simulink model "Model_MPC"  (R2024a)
settings: Solver=VariableStepAuto  StartTime=0.0  StopTime=10.0  RelTol=1e-3
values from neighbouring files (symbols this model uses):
  A_f = 2.15    [main.m]    (also in prediction_longitudinal_model.m; MPC_and_plant_params.m; prediction_model_test.m; main_BW_FW.m)
  alpha = 0*pi/180    (= 0)    [main.m]    (also in prediction_longitudinal_model.m; MPC_and_plant_params.m; prediction_model_test.m; main_BW_FW.m)
  C_d = 0.33    [main.m]    (also in prediction_longitudinal_model.m; MPC_and_plant_params.m; prediction_model_test.m; main_BW_FW.m)
  default_distance = 10    [main.m]    (also in MPC_and_plant_params.m = 50)
  eff = e    [polinomial_fits.m]    (also in eff_poly.m; main.m = Efficiency/100; MPC_and_plant_params.m = Efficiency/100; main_BW_FW.m = Efficiency/100)
  f_0 = 4.5*1e-3    (= 0.0045)    [main.m]    (also in prediction_longitudinal_model.m; MPC_and_plant_params.m; prediction_model_test.m; main_BW_FW.m)
  g = 9.81    [main.m]    (also in prediction_longitudinal_model.m; MPC_and_plant_params.m; prediction_model_test.m; main_BW_FW.m)
  h = 0.3    [main.m]    (also in prediction_longitudinal_model.m; MPC_and_plant_params.m = 2; main_BW_FW.m)
  K = nmpc_design_4b(par)    [main.m]
  lambda = 0.5    [main.m]    (also in MPC_and_plant_params.m)
  M_veh = 1400    [main.m]    (also in prediction_longitudinal_model.m; MPC_and_plant_params.m; prediction_model_test.m; main_BW_FW.m)
  max_acc = 2    [main.m]    (also in MPC_and_plant_params.m)
  min_acc = -3    [main.m]    (also in MPC_and_plant_params.m)
  N_p = 1    [main.m]    (also in prediction_longitudinal_model.m; MPC_and_plant_params.m; prediction_model_test.m; main_BW_FW.m)
  N_s = 108    [main.m]    (also in prediction_longitudinal_model.m; MPC_and_plant_params.m; prediction_model_test.m; main_BW_FW.m)
  r_w = 0.3    [main.m]    (also in prediction_longitudinal_model.m; MPC_and_plant_params.m; prediction_model_test.m; main_BW_FW.m)
  ref_mode = 3    [main.m]
  rho = 1.25    [main.m]    (also in prediction_longitudinal_model.m; MPC_and_plant_params.m; prediction_model_test.m; main_BW_FW.m)
  Ro_s = F_Ro_s(SOC_vec)    [main.m]    (also in MPC_and_plant_params.m; main_BW_FW.m)
  s = tf('s')    [main.m]    (also in MPC_and_plant_params.m; polinomial_fits.m = size(Speed))
  SOC0 = 0.8    [main.m]    (also in MPC_and_plant_params.m; prediction_model_test.m; main_BW_FW.m)
  SOC_vec = linspace(0,1,500)    [main.m]    (also in MPC_and_plant_params.m; main_BW_FW.m)
  tau_gb = 9.6    [main.m]    (also in prediction_longitudinal_model.m; MPC_and_plant_params.m; prediction_model_test.m; main_BW_FW.m)
  time_gap = 3    [main.m]    (also in MPC_and_plant_params.m)
  Ts = 0.05    [main.m]    (also in MPC_and_plant_params.m)
  v0 = vehspeed(1)    [main.m]    (also in MPC_and_plant_params.m; prediction_model_test.m = 0)
  v_set = 40    [main.m]    (also in MPC_and_plant_params.m)
  verr_gain = 0.1    [main.m]    (also in MPC_and_plant_params.m)
  Voc_s = F_Voc_s(SOC_vec)    [main.m]    (also in MPC_and_plant_params.m; main_BW_FW.m)
  vx_gain = 0.5    [main.m]    (also in MPC_and_plant_params.m)
  x0 = 0    [main.m]    (also in MPC_and_plant_params.m; prediction_model_test.m)
  xerr_gain = 0.3    [main.m]    (also in MPC_and_plant_params.m)
undefined symbols (not defined in the file or in its folder): flip, m, seconds, Shaft_Torque, Speed
libraries: slpidlib x2, autolibshared x1, cstblocks x1

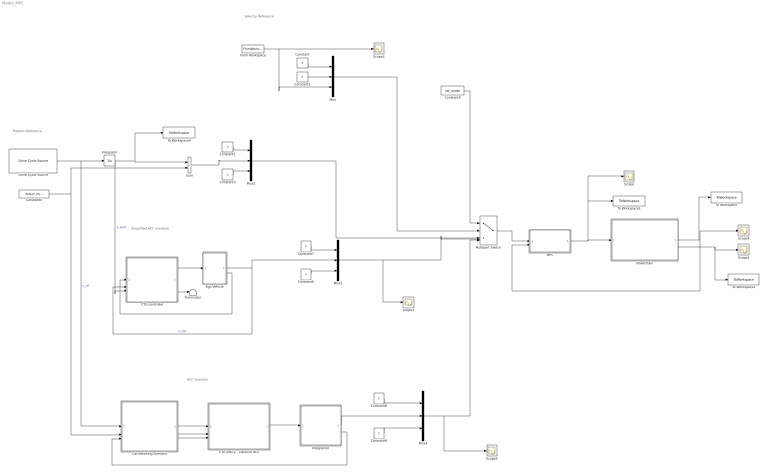
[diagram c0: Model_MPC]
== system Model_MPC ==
  note: Velocity Reference
  note: Position Reference
  note: Simplified ACC Scenario
  note: ACC Scenario
  CTG controller : Subsystem
  CTG policy - classical ACC : Subsystem  Commented=on
  Car-following Scenario : Subsystem  Commented=on
  Constant{,1..3,8..9} (6 alike) : Constant  Commented=on  Value=0
  Constant4 : Constant  Value=default_distance
  Constant5 : Constant  Value=ref_mode
  Constant6 : Constant  Value=0
  Constant7 : Constant  Value=0
  Drive Cycle Source : autolibshared/Drive Cycle Source  cycleVar=Workspace variable  wsVar=vehspeed  fileVar=cycleFTP75.mat  tfinal="1800  seconds"  cycleRepeat=off  outAccPort=off  outGearPort=off  gearList=No gear data  t_wot1=5  xdot_woto=0  xdot_wot1=30  t_wot2=20  xdot_wot2=0  t_wotend=30  srcUnit=m/s  outUnit=m/s  srcAccUnit=m/s/s  outAccUnit=m/s^2  dt=0  aMode=1  faultOption=off  velBnd=2  velBndUnit=mph  inUnit=m/s  timeBnd=1  failOption=off  stopSim=off  maxFaultCnt=10  maxFaultTime=2  maxTotFaultTime=15  traceOption=off  dtTrace=1  traceWindow=10  lastDCname=Custom Data Set  lastOutUnit=mph  lastDT=0  lastTB=1  lastSB=2  forceCalcBound=off
  Ego Vehicle : Subsystem
  From Workspace : FromWorkspace  Commented=on  VariableName=vehspeed  SampleTime=0.1  OutputAfterFinalValue=Holding final value
  Integration : Subsystem  Commented=on
  Integrator : Integrator  InitialCondition=default_distance
  MPC : Subsystem
  Multiport Switch : MultiPortSwitch  Inputs=4
  Mux : Mux  Commented=on  Inputs=3
  Mux1 : Mux  Commented=on  Inputs=3
  Mux2 : Mux  Inputs=3
  Mux3 : Mux  Commented=on  Inputs=3
  Powertrain : Subsystem
  Scope{,1..5} (6 alike) : Scope
  Sum : Sum  Commented=on  Inputs=+-
  Terminator : Terminator
  To Workspace : ToWorkspace  VariableName=X  SaveFormat=Timeseries  SampleTime=-1
  To Workspace1 : ToWorkspace  VariableName=T_EM_MPC  SaveFormat=Timeseries  SampleTime=-1
  To Workspace2 : ToWorkspace  VariableName=X_dot  SaveFormat=Timeseries  SampleTime=-1
  To Workspace4 : ToWorkspace  VariableName=pos_leading  SaveFormat=Timeseries  SampleTime=-1
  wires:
  MPC/1(u) -> Powertrain/1(T_EM), To Workspace1/1, Scope/1
  Powertrain/1(X (states)) -> To Workspace/1, MPC/2(x), Scope4/1
  Powertrain/2(X_dot) -> To Workspace2/1, Scope1/1
  From Workspace/1 -> Mux/3, Scope2/1
  Constant2/1 -> Mux/2
  Constant/1 -> Mux/1
  Drive Cycle Source/1 -> Car-following Scenario/1(lead speed [m/s]), Integrator/1  "v_ref"
  Constant1/1 -> Mux1/1
  Constant3/1 -> Mux1/3
  Integrator/1 -> To Workspace4/1, Sum/1, CTG controller/3(lead position [m])  "x_lead"
  Constant4/1 -> Car-following Scenario/2(initial distance [m]), Sum/2
  CTG controller/1(a) -> Ego Vehicle/1(a)
  Ego Vehicle/1(x) -> CTG controller/2(ego position [m]), Mux2/2  "x_ego"
  Constant7/1 -> Mux2/1
  Constant6/1 -> Mux2/3
  CTG controller/2(spacing_error) -> Terminator/1
  Multiport Switch/1 -> MPC/1(r)
  Constant5/1 -> Multiport Switch/1
  Mux1/1 -> Multiport Switch/3
  Mux2/1 -> Scope3/1, Multiport Switch/4
  Ego Vehicle/2(x_dot) -> CTG controller/1(ego speed [m/s])
  Car-following Scenario/1(d_rel) -> CTG policy - classical ACC/1(Relative Distance)
  Car-following Scenario/2(v_rel) -> CTG policy - classical ACC/2("Relative Velocity ")
  Car-following Scenario/3(v_host) -> CTG policy - classical ACC/3("Longitudinal Velocity ")
  Constant8/1 -> Mux3/1
  Constant9/1 -> Mux3/3
  Mux3/1 -> Scope5/1, Multiport Switch/5
  Sum/1 -> Mux1/2
  Mux/1 -> Multiport Switch/2
  Integration/1(x_ego) -> Mux3/2
  CTG policy - classical ACC/1(Acceleration) -> Integration/1(a)
  Integration/2(x_dot) -> Car-following Scenario/3(ego speed [m/s])

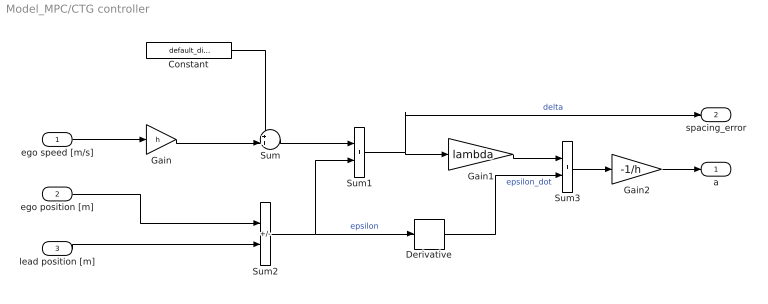
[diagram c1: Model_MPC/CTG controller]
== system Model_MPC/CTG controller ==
  ego speed [m/s] : Inport
  ego position [m] : Inport  Port=2
  lead position [m] : Inport  Port=3
  Constant : Constant  Value=default_distance
  Derivative : Derivative  CoefficientInTFapproximation=Td
  Gain : Gain  Gain=h
  Gain1 : Gain  Gain=lambda
  Gain2 : Gain  Gain=-1/h
  Sum : Sum  Inputs=++|
  Sum1 : Sum
  Sum2 : Sum  Inputs=+-
  Sum3 : Sum
  a : Outport
  spacing_error : Outport  Port=2
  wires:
  ego position [m]/1 -> Sum2/1
  lead position [m]/1 -> Sum2/2
  ego speed [m/s]/1 -> Gain/1
  Sum2/1 -> Derivative/1, Sum1/2  "epsilon"
  Sum1/1 -> spacing_error/1, Gain1/1  "delta"
  Sum3/1 -> Gain2/1
  Derivative/1 -> Sum3/2  "epsilon_dot"
  Gain1/1 -> Sum3/1
  Gain2/1 -> a/1
  Gain/1 -> Sum/2
  Sum/1 -> Sum1/1
  Constant/1 -> Sum/1

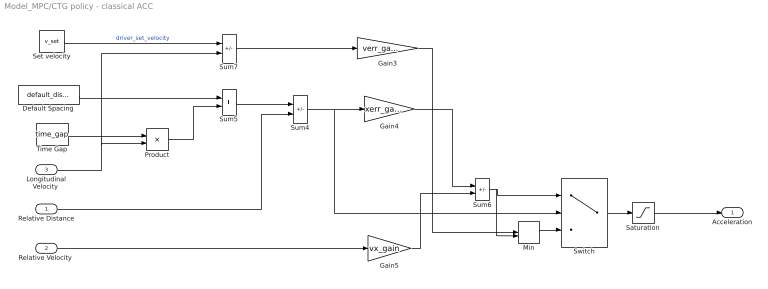
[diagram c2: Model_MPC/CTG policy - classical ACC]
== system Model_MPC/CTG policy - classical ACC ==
  Relative Distance : Inport
  "Relative Velocity " : Inport  Port=2
  "Longitudinal Velocity " : Inport  Port=3
  Default Spacing : Constant  Value=default_distance  SampleTime=Ts
  Gain3 : Gain  Gain=verr_gain
  Gain4 : Gain  Gain=xerr_gain
  Gain5 : Gain  Gain=vx_gain
  Min : MinMax  Inputs=2
  Product : Product
  Saturation : Saturate  UpperLimit=max_acc  LowerLimit=min_acc
  Set velocity : Constant  Value=v_set  SampleTime=Ts
  Sum4 : Sum  Inputs=+-
  Sum5 : Sum
  Sum6 : Sum  Inputs=-+
  Sum7 : Sum  Inputs=+-
  Switch : Switch  Criteria=u2 > Threshold
  Time Gap : Constant  Value=time_gap  SampleTime=Ts
  Acceleration : Outport  VectorParamsAs1DForOutWhenUnconnected=off
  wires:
  Sum6/1 -> Min/2, Switch/1
  Sum5/1 -> Sum4/1
  Saturation/1 -> Acceleration/1
  Min/1 -> Switch/3
  "Longitudinal Velocity "/1 -> Sum7/2, Product/2
  Set velocity/1 -> Sum7/1  "driver_set_velocity"
  Time Gap/1 -> Product/1
  Gain3/1 -> Min/1
  Relative Distance/1 -> Sum4/2
  Gain4/1 -> Sum6/1
  "Relative Velocity "/1 -> Gain5/1
  Product/1 -> Sum5/2
  Switch/1 -> Saturation/1
  Gain5/1 -> Sum6/2
  Sum7/1 -> Gain3/1
  Sum4/1 -> Switch/2, Gain4/1
  Default Spacing/1 -> Sum5/1

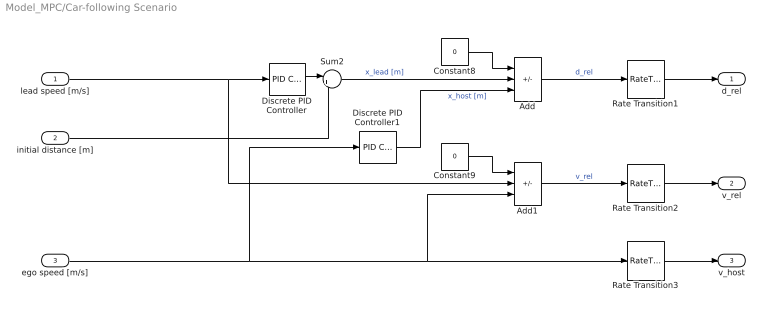
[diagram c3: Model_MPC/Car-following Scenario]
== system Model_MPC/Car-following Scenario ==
  lead speed [m/s] : Inport
  initial distance [m] : Inport  Port=2
  ego speed [m/s] : Inport  Port=3
  Add : Sum  Inputs=++-
  Add1 : Sum  Inputs=++-
  Constant8 : Constant  Value=0
  Constant9 : Constant  Value=0
  Discrete PID Controller : slpidlib/PID Controller  Controller=I  Form=Parallel  TimeDomain=Discrete-time  UseExternalTs=off  SampleTime=-1  IntegratorMethod=Forward Euler  FilterMethod=Forward Euler  ControllerParametersSource=internal  P=0  I=1  UseKiTs=off  D=0  UseExternalDerivativeSource=off  N=100  UseFilter=on  TunerSelectOption=Transfer Function Based (PID Tuner App)  InitialConditionSource=internal  InitialConditionForIntegrator=0  InitialConditionForFilter=0  DifferentiatorICPrevScaledInput=0  ExternalReset=none  TrackingMode=off  Kt=1  LimitOutput=off  SatLimitsSource=internal  UpperSaturationLimit=inf  LowerSaturationLimit=-inf  LinearizeAsGain=off  AntiWindupMode=none  Kb=1  LimitIntegrator=off  UpperIntegratorSaturationLimit=inf  LowerIntegratorSaturationLimit=-inf  POutMin=[]  POutMax=[]  IOutMin=[]  IOutMax=[]  DOutMin=[]  DOutMax=[]  NOutMin=[]  NOutMax=[]  SumOutMin=[]  SumOutMax=[]  SaturationOutMin=[]  SaturationOutMax=[]  PParamMin=[]  PParamMax=[]  IParamMin=[]  IParamMax=[]  DParamMin=[]  DParamMax=[]  NParamMin=[]  NParamMax=[]  KbParamMin=[]  KbParamMax=[]  KtParamMin=[]  KtParamMax=[]  KbOutMin=[]  KbOutMax=[]  KtOutMin=[]  KtOutMax=[]  IntegratorOutMin=[]  IntegratorOutMax=[]  FilterOutMin=[]  FilterOutMax=[]  SumI1OutMin=[]  SumI1OutMax=[]  SumI2OutMin=[]  SumI2OutMax=[]  SumI3OutMin=[]  SumI3OutMax=[]  SumI4OutMin=[]  SumI4OutMax=[]  SumDOutMin=[]  SumDOutMax=[]  DifferentiatorOutMin=[]  DifferentiatorOutMax=[]  FilterDiffOutCoefMin=[]  FilterDiffOutCoefMax=[]  ReciprocalOutMin=[]  ReciprocalOutMax=[]  SumDenOutMin=[]  SumDenOutMax=[]  SumNumOutMin=[]  SumNumOutMax=[]  DivideOutMin=[]  DivideOutMax=[]  UdiffTsProdOutMin=[]  UdiffTsProdOutMax=[]  NTsProdOutMin=[]  NTsProdOutMax=[]  UintegralTsProdOutMin=[]  UintegralTsProdOutMax=[]  UngainTsProdOutMin=[]  UngainTsProdOutMax=[]  ClampingZeroOutDataTypeStr=Inherit: Inherit via back propagation  ClampingZeroOutMin=[]  ClampingZeroOutMax=[]  FilterDenConstantOutDataTypeStr=Inherit: Inherit via back propagation  FilterDenConstantOutMin=[]  FilterDenConstantOutMax=[]  PCopyOutDataTypeStr=Inherit: Inherit via back propagation  PCopyOutMin=[]  PCopyOutMax=[]  NCopyOutDataTypeStr=Inherit: Inherit via back propagation  NCopyOutMin=[]  NCopyOutMax=[]  IntegratorContinuousStateAttributes=''  IntegratorStateMustResolveToSignalObject=off  IntegratorRTWStateStorageClass=Auto  FilterContinuousStateAttributes=''  FilterStateMustResolveToSignalObject=off  FilterRTWStateStorageClass=Auto  ParallelPVariant=Disabled  IdealPVariant=Disabled  IVariant=InternalParameters  DVariant=Disabled  IntegratorVariant=Discrete  SatVariant=Disabled  AWVariant=Passthrough  PCopyVariant=Disabled  TRVariant=Disabled  FdbkBlocksVariant=Forward  IdealPFdbkVariant=Disabled  SatFdbkVariant=Disabled  DerivativeFilterVariant=Disabled  NVariant=Disabled  NCopyVariant=Disabled_SignalSpec  FilterICVariant=Disabled  IntegratorICVariant=InternalICs  ExternalResetVariant=Disabled  TRSumVariant=Passthrough  SumFdbkVariant=Disabled  SumVariant=Passthrough_I  TsampFilterVariant=InternalTs  TsampNgainVariant=Passthrough  TsampIntegralVariant=Disabled_SignalSpec  ExternalSaturationOutDataTypeStr=Inherit: Same as second input  DerivativeSourceVariant=Disabled
  Discrete PID Controller1 : slpidlib/PID Controller  Controller=I  Form=Parallel  TimeDomain=Discrete-time  UseExternalTs=off  SampleTime=-1  IntegratorMethod=Forward Euler  FilterMethod=Forward Euler  ControllerParametersSource=internal  P=0  I=1  UseKiTs=off  D=0  UseExternalDerivativeSource=off  N=100  UseFilter=on  TunerSelectOption=Transfer Function Based (PID Tuner App)  InitialConditionSource=internal  InitialConditionForIntegrator=0  InitialConditionForFilter=0  DifferentiatorICPrevScaledInput=0  ExternalReset=none  TrackingMode=off  Kt=1  LimitOutput=off  SatLimitsSource=internal  UpperSaturationLimit=inf  LowerSaturationLimit=-inf  LinearizeAsGain=off  AntiWindupMode=none  Kb=1  LimitIntegrator=off  UpperIntegratorSaturationLimit=inf  LowerIntegratorSaturationLimit=-inf  POutMin=[]  POutMax=[]  IOutMin=[]  IOutMax=[]  DOutMin=[]  DOutMax=[]  NOutMin=[]  NOutMax=[]  SumOutMin=[]  SumOutMax=[]  SaturationOutMin=[]  SaturationOutMax=[]  PParamMin=[]  PParamMax=[]  IParamMin=[]  IParamMax=[]  DParamMin=[]  DParamMax=[]  NParamMin=[]  NParamMax=[]  KbParamMin=[]  KbParamMax=[]  KtParamMin=[]  KtParamMax=[]  KbOutMin=[]  KbOutMax=[]  KtOutMin=[]  KtOutMax=[]  IntegratorOutMin=[]  IntegratorOutMax=[]  FilterOutMin=[]  FilterOutMax=[]  SumI1OutMin=[]  SumI1OutMax=[]  SumI2OutMin=[]  SumI2OutMax=[]  SumI3OutMin=[]  SumI3OutMax=[]  SumI4OutMin=[]  SumI4OutMax=[]  SumDOutMin=[]  SumDOutMax=[]  DifferentiatorOutMin=[]  DifferentiatorOutMax=[]  FilterDiffOutCoefMin=[]  FilterDiffOutCoefMax=[]  ReciprocalOutMin=[]  ReciprocalOutMax=[]  SumDenOutMin=[]  SumDenOutMax=[]  SumNumOutMin=[]  SumNumOutMax=[]  DivideOutMin=[]  DivideOutMax=[]  UdiffTsProdOutMin=[]  UdiffTsProdOutMax=[]  NTsProdOutMin=[]  NTsProdOutMax=[]  UintegralTsProdOutMin=[]  UintegralTsProdOutMax=[]  UngainTsProdOutMin=[]  UngainTsProdOutMax=[]  ClampingZeroOutDataTypeStr=Inherit: Inherit via back propagation  ClampingZeroOutMin=[]  ClampingZeroOutMax=[]  FilterDenConstantOutDataTypeStr=Inherit: Inherit via back propagation  FilterDenConstantOutMin=[]  FilterDenConstantOutMax=[]  PCopyOutDataTypeStr=Inherit: Inherit via back propagation  PCopyOutMin=[]  PCopyOutMax=[]  NCopyOutDataTypeStr=Inherit: Inherit via back propagation  NCopyOutMin=[]  NCopyOutMax=[]  IntegratorContinuousStateAttributes=''  IntegratorStateMustResolveToSignalObject=off  IntegratorRTWStateStorageClass=Auto  FilterContinuousStateAttributes=''  FilterStateMustResolveToSignalObject=off  FilterRTWStateStorageClass=Auto  ParallelPVariant=Disabled  IdealPVariant=Disabled  IVariant=InternalParameters  DVariant=Disabled  IntegratorVariant=Discrete  SatVariant=Disabled  AWVariant=Passthrough  PCopyVariant=Disabled  TRVariant=Disabled  FdbkBlocksVariant=Forward  IdealPFdbkVariant=Disabled  SatFdbkVariant=Disabled  DerivativeFilterVariant=Disabled  NVariant=Disabled  NCopyVariant=Disabled_SignalSpec  FilterICVariant=Disabled  IntegratorICVariant=InternalICs  ExternalResetVariant=Disabled  TRSumVariant=Passthrough  SumFdbkVariant=Disabled  SumVariant=Passthrough_I  TsampFilterVariant=InternalTs  TsampNgainVariant=Passthrough  TsampIntegralVariant=Disabled_SignalSpec  ExternalSaturationOutDataTypeStr=Inherit: Same as second input  DerivativeSourceVariant=Disabled
  Rate Transition1 : RateTransition  OutPortSampleTime=0.2
  Rate Transition2 : RateTransition  OutPortSampleTime=0.2
  Rate Transition3 : RateTransition  OutPortSampleTime=0.2
  Sum2 : Sum  Inputs=|++
  d_rel : Outport
  v_rel : Outport  Port=2
  v_host : Outport  Port=3
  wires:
  initial distance [m]/1 -> Sum2/2
  Rate Transition1/1 -> d_rel/1
  Rate Transition2/1 -> v_rel/1
  ego speed [m/s]/1 -> Discrete PID Controller1/1, Add1/3, Rate Transition3/1
  Constant8/1 -> Add/1
  lead speed [m/s]/1 -> Add1/2, Discrete PID Controller/1
  Constant9/1 -> Add1/1
  Discrete PID Controller/1 -> Sum2/1
  Discrete PID Controller1/1 -> Add/3  "x_host [m]"
  Add1/1 -> Rate Transition2/1  "v_rel"
  Rate Transition3/1 -> v_host/1
  Add/1 -> Rate Transition1/1  "d_rel"
  Sum2/1 -> Add/2  "x_lead [m]"

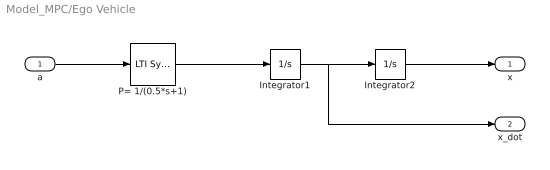
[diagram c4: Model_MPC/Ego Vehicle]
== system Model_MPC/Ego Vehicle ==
  a : Inport
  Integrator1 : Integrator
  Integrator2 : Integrator
  P= 1/(0.5*s+1) : cstblocks/LTI System  sys=P  IC=[]  PadeOrder=0
  x : Outport
  x_dot : Outport  Port=2
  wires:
  Integrator2/1 -> x/1
  Integrator1/1 -> x_dot/1, Integrator2/1
  P= 1/(0.5*s+1)/1 -> Integrator1/1
  a/1 -> P= 1/(0.5*s+1)/1

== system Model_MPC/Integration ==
  a : Inport
  Integrator1 : Integrator
  Integrator2 : Integrator
  x_ego : Outport
  x_dot : Outport  Port=2
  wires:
  Integrator2/1 -> x_ego/1  "x_ego"
  a/1 -> Integrator1/1
  Integrator1/1 -> x_dot/1, Integrator2/1

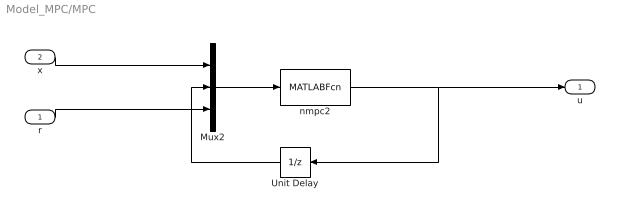
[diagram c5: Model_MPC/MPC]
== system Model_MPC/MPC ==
  r : Inport
  x : Inport  Port=2
  Mux2 : Mux  Inputs=3
  Unit Delay : UnitDelay  InitialCondition=zeros(K.nc,1)  SampleTime=K.Ts  HasFrameUpgradeWarning=on
  nmpc2 : MATLABFcn  MATLABFcn=nmpc_b2(K,u(1:K.nx),u(K.nx+1:K.nx+K.nc),u(K.nx+K.nc+1:end))  OutputDimensions=K.nc
  u : Outport
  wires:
  x/1 -> Mux2/1
  r/1 -> Mux2/3
  Unit Delay/1 -> Mux2/2
  Mux2/1 -> nmpc2/1
  nmpc2/1 -> Unit Delay/1, u/1

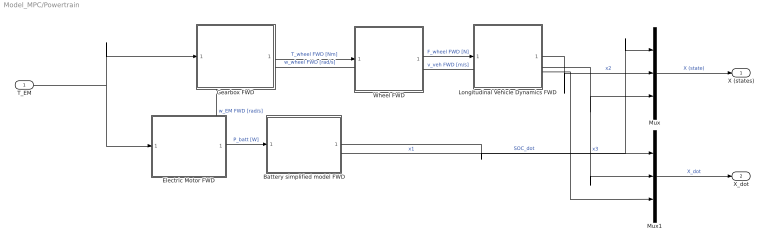
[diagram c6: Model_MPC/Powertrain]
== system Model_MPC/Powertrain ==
  T_EM : Inport
  Battery simplified model FWD : Subsystem
  Electric Motor FWD : Subsystem
  Gearbox FWD : Subsystem
  Longitudinal Vehicle Dynamics FWD : Subsystem
  Mux : Mux  Inputs=3
  Mux1 : Mux  Inputs=3
  Wheel FWD : Subsystem
  X (states) : Outport
  X_dot : Outport  Port=2
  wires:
  Battery simplified model FWD/2(SOC) -> Mux/1  "x1"
  Wheel FWD/2(w_wheel) -> Gearbox FWD/2(w_wheel)  "w_wheel FWD [rad/s]"
  Mux/1 -> X (states)/1  "X (state)"
  Gearbox FWD/1(T_wheel) -> Wheel FWD/1(T_wheel)  "T_wheel FWD [Nm]"
  Longitudinal Vehicle Dynamics FWD/2(v_veh) -> Mux1/2, Mux/3  "x3"
  Gearbox FWD/2(w_EM) -> Electric Motor FWD/2(w_EM)  "w_EM FWD [rad/s]"
  Electric Motor FWD/1(P_batt) -> Battery simplified model FWD/1(P_batt)  "P_batt [W]"
  Longitudinal Vehicle Dynamics FWD/4(v_veh1) -> Wheel FWD/2(v_veh)  "v_veh FWD [m/s]"
  Longitudinal Vehicle Dynamics FWD/1("x_veh ") -> Mux/2  "x2"
  Wheel FWD/1(F_wheel) -> Longitudinal Vehicle Dynamics FWD/1(F_trac)  "F_wheel FWD [N]"
  T_EM/1 -> Electric Motor FWD/1(T_EM), Gearbox FWD/1(T_EM)
  Battery simplified model FWD/1(SOC_dot) -> Mux1/1  "SOC_dot"
  Longitudinal Vehicle Dynamics FWD/3(a_veh) -> Mux1/3
  Mux1/1 -> X_dot/1  "X_dot"

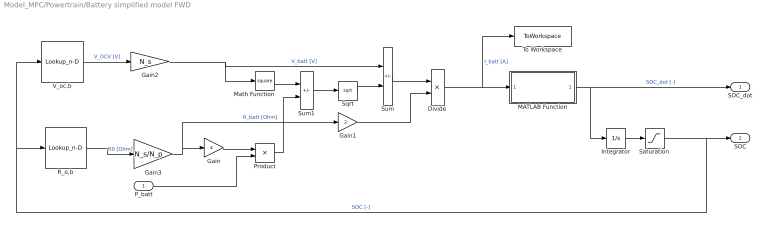
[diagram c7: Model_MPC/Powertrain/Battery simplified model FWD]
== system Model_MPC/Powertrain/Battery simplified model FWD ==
  P_batt : Inport
  Divide : Product  Inputs=*/
  Gain : Gain  Gain=4
  Gain1 : Gain  Gain=2
  Gain2 : Gain  Gain=N_s
  Gain3 : Gain  Gain=N_s/N_p
  Integrator : Integrator  InitialCondition=SOC0
  MATLAB Function : MATLAB Function  TreatAsAtomicUnit=on
  Math Function : Math  Operator=square
  Product : Product
  R_o,b : Lookup_n-D  NumberOfTableDimensions=1  BreakpointsForDimension1=SOC_vec  BreakpointsForDimension3=[5, 7]  Table=Ro_s  InternalRulePriority=Speed  RndMeth=Simplest
  Saturation : Saturate  UpperLimit=1  LowerLimit=0
  Sqrt : Sqrt
  Sum : Sum  Inputs=+-
  Sum1 : Sum  Inputs=+-
  To Workspace : ToWorkspace  VariableName=Ib_controlled  SaveFormat=Timeseries  SampleTime=-1
  V_oc,b : Lookup_n-D  NumberOfTableDimensions=1  BreakpointsForDimension1=SOC_vec  BreakpointsForDimension3=[5, 7]  Table=Voc_s  InternalRulePriority=Speed  RndMeth=Simplest
  SOC_dot : Outport
  SOC : Outport  Port=2
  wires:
  Math Function/1 -> Sum1/1
  Gain/1 -> Product/1
  Product/1 -> Sum1/2
  Sum1/1 -> Sqrt/1
  Sqrt/1 -> Sum/2
  Sum/1 -> Divide/1
  Gain1/1 -> Divide/2
  Divide/1 -> MATLAB Function/1(I_b), To Workspace/1  "I_batt [A]"
  MATLAB Function/1(SOC_dot) -> SOC_dot/1, Integrator/1  "SOC_dot [-]"
  Integrator/1 -> Saturation/1
  R_o,b/1 -> Gain3/1  "R0 [Ohm]"
  V_oc,b/1 -> Gain2/1  "V_OCV [V]"
  Gain2/1 -> Sum/1, Math Function/1  "V_batt [V]"
  Gain3/1 -> Gain1/1, Gain/1  "R_batt [Ohm]"
  Saturation/1 -> R_o,b/1, V_oc,b/1, SOC/1  "SOC [-]"
  P_batt/1 -> Product/2

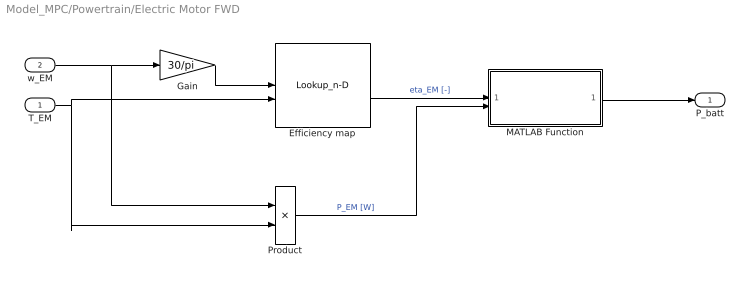
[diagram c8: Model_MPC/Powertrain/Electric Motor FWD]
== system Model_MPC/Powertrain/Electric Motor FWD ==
  T_EM : Inport
  w_EM : Inport  Port=2
  Efficiency map : Lookup_n-D  BreakpointsForDimension1=Speed(:,1)  BreakpointsForDimension2=flip(Shaft_Torque(1,:))  BreakpointsForDimension3=[5, 7]  Table=flip(eff)  InternalRulePriority=Speed  RndMeth=Simplest
  Gain : Gain  Gain=30/pi
  MATLAB Function : MATLAB Function  TreatAsAtomicUnit=on
  Product : Product
  P_batt : Outport
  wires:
  w_EM/1 -> Gain/1, Product/1
  T_EM/1 -> Efficiency map/2, Product/2
  Product/1 -> MATLAB Function/2(P_EM)  "P_EM [W]"
  MATLAB Function/1(P_batt) -> P_batt/1
  Efficiency map/1 -> MATLAB Function/1(eta_EM)  "eta_EM [-]"
  Gain/1 -> Efficiency map/1

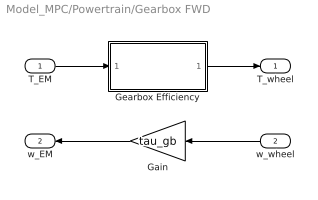
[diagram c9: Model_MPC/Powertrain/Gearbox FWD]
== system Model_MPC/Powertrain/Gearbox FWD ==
  T_EM : Inport
  w_wheel : Inport  Port=2
  Gain : Gain  Gain=tau_gb
  Gearbox Efficiency : MATLAB Function  TreatAsAtomicUnit=on
  T_wheel : Outport
  w_EM : Outport  Port=2
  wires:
  T_EM/1 -> Gearbox Efficiency/1(T_EM)
  Gearbox Efficiency/1(T_wheel) -> T_wheel/1
  w_wheel/1 -> Gain/1
  Gain/1 -> w_EM/1

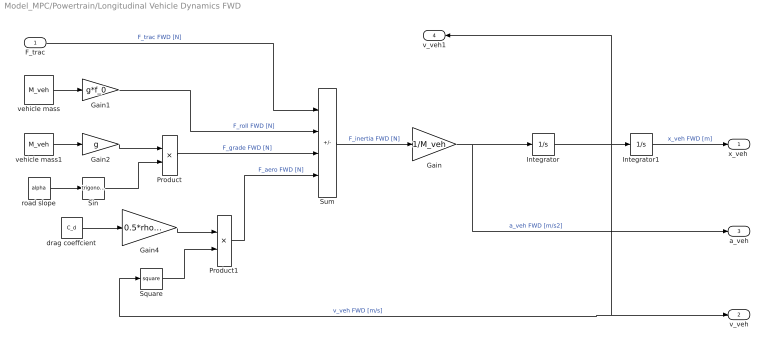
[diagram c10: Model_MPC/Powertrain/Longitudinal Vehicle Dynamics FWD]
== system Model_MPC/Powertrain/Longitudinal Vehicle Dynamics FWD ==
  F_trac : Inport
  Gain : Gain  Gain=1/M_veh
  Gain1 : Gain  Gain=g*f_0
  Gain2 : Gain  Gain=g
  Gain4 : Gain  Gain=0.5*rho*A_f
  Integrator : Integrator  InitialCondition=v0
  Integrator1 : Integrator  InitialCondition=x0
  Product : Product
  Product1 : Product
  Sin : Trigonometry
  Square : Math  Operator=square
  Sum : Sum  Inputs=+---
  drag coeffcient : Constant  Value=C_d
  road slope : Constant  Value=alpha
  vehicle mass : Constant  Value=M_veh
  vehicle mass1 : Constant  Value=M_veh
  "x_veh " : Outport
  v_veh : Outport  Port=2
  a_veh : Outport  Port=3
  v_veh1 : Outport  Port=4
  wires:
  drag coeffcient/1 -> Gain4/1
  Gain2/1 -> Product/1
  vehicle mass/1 -> Gain1/1
  Gain1/1 -> Sum/2  "F_roll FWD [N]"
  vehicle mass1/1 -> Gain2/1
  road slope/1 -> Sin/1
  Product1/1 -> Sum/4  "F_aero FWD [N]"
  Sin/1 -> Product/2
  Product/1 -> Sum/3  "F_grade FWD [N]"
  F_trac/1 -> Sum/1  "F_trac FWD [N]"
  Gain4/1 -> Product1/1
  Square/1 -> Product1/2
  Sum/1 -> Gain/1  "F_inertia FWD [N]"
  Gain/1 -> a_veh/1, Integrator/1  "a_veh FWD [m/s2]"
  Integrator/1 -> Square/1, v_veh/1, v_veh1/1, Integrator1/1  "v_veh FWD [m/s]"
  Integrator1/1 -> "x_veh "/1  "x_veh FWD [m]"

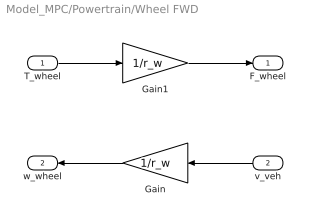
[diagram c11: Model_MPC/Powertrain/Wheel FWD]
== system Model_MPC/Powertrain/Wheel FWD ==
  T_wheel : Inport
  v_veh : Inport  Port=2
  Gain : Gain  Gain=1/r_w
  Gain1 : Gain  Gain=1/r_w
  F_wheel : Outport
  w_wheel : Outport  Port=2
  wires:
  T_wheel/1 -> Gain1/1
  Gain1/1 -> F_wheel/1
  v_veh/1 -> Gain/1
  Gain/1 -> w_wheel/1

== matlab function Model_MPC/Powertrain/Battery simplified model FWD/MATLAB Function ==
function SOC_dot = fcn(I_b)
    eta_c = 0.95;
    Q_nom = 60*1*3600;
    if I_b > 0 % discharge
        SOC_dot = -I_b/(eta_c*Q_nom);
    else % charge
        SOC_dot = -eta_c*I_b/Q_nom;
    end

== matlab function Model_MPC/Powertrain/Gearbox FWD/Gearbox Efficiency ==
function T_wheel = fcn(T_EM)
eta_gb = 0.97;
tau_gb = 9.6;

T_wheel = T_EM * ((tau_gb*eta_gb^(sign(T_EM))));
% T_wheel = T_EM*tau_gb;

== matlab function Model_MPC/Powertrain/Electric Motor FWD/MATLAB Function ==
function P_batt = fcn(eta_EM,P_EM)
eta_inv = 1;

P_batt = P_EM/((eta_EM*eta_inv)^(sign(P_EM)));  
% P_batt = P_EM/(eta_EM*eta_inv);
